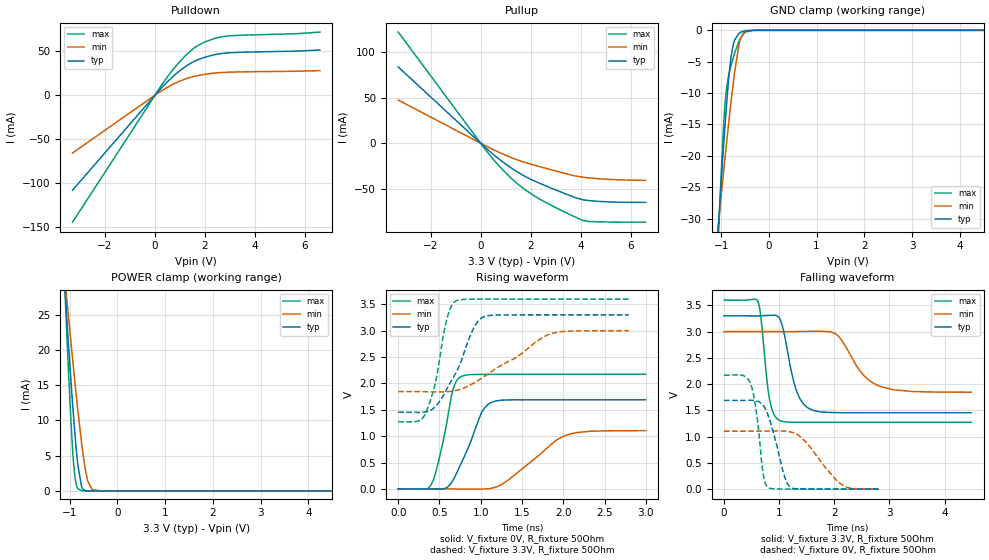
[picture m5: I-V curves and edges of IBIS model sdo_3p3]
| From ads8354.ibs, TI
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|   sdo_3p3 Model
[Model]   sdo_3p3
Model_type   3-state
Polarity   Non-Inverting
Vmeas = 1.65
Vref = 0
Cref = 10pF
Rref = 100
|   typ   min   max
|   (nom PVT)   (fast PVT)   (slow PVT)
C_comp   1.168e-12   9.199e-13   1.410e-12
| Where nom  PVT is Nominal Process, 3.3V, 27C
|   Fast PVT is Strong Process,  3.6V, -40C
|   Slow PVT is Weak Process,   3V, 125C
[Voltage Range]   3.3   3   3.6
|Junction Temperature
[Temperature Range]   27   125   -40
[Pullup Reference]   3.3   3   3.6
[Pulldown Reference]   0   0   0
[Power Clamp Reference]   3.3   3   3.6
[GND Clamp Reference]   0   0   0
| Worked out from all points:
|   slope of the pulldown table from 0 to 0.495 V, typ, clamps not added: 32.3 ohm
|   slope of the pullup table from 0 to 0.495 V, typ, clamps not added: 41.1 ohm
|   GND clamp passes 1 mA (typ) near -0.67 V on its own axis
|   POWER clamp passes 1 mA (typ) near -0.76 V on its own axis
|   falling waveform, V_fixture 3.3V, R_fixture 50Ohm: 20-80 % time 236ps typ, 455ps min, 138ps max; typ from 3.3 V to 1.45 V
|   rising waveform, V_fixture 0V, R_fixture 50Ohm: 20-80 % time 266ps typ, 510ps min, 168ps max; typ from 0 V to 1.69 V
|   rising waveform, V_fixture 3.3V, R_fixture 50Ohm: 20-80 % time 314ps typ, 664ps min, 173ps max; typ from 1.45 V to 3.3 V
|   falling waveform, V_fixture 0V, R_fixture 50Ohm: 20-80 % time 253ps typ, 496ps min, 146ps max; typ from 1.69 V to 0 V
[Pulldown]
|   Voltage   I(typ)   I(min)   I(max)
-3.3V     -108.3mA   -65.93mA   -144.9mA
276mV     8.889mA    5.263mA    12.04mA
580.8mV   17.73mA    10.37mA    24.11mA
922.8mV   26.37mA    15.19mA    36.09mA
1.254V    33.38mA    18.88mA    46.05mA
1.582V    38.81mA    21.55mA    54.12mA
1.833V    41.77mA    23.03mA    58.51mA
2.262V    45.4mA     24.87mA    63.57mA
2.835V    48.1mA     26.13mA    67.38mA
5.702V    50.35mA    27.36mA    70.25mA
6.6V      51.63mA    28.07mA    72.02mA
[GND Clamp]
|   Voltage   I(typ)   I(min)   I(max)
-3.3V     -330.2mA   -221.1mA   -504.8mA
-1.063V   -31.82mA   -31.36mA   -34mA
-1.01V    -25.58mA   -27.31mA   -24.71mA
-943.8mV  -17.95mA   -22.25mA   -14.61mA
-921mV    -15.46mA   -20.55mA   -12mA
-881.1mV  -11.36mA   -17.62mA   -8.898mA
-788.7mV  -4.041mA   -11.17mA   -5.539mA
-745.8mV  -2.266mA   -8.406mA   -4.364mA
-624mV    -483.8uA   -2.208mA   -1.712mA
-528mV    -102.4uA   -293.2uA   -540.5uA
-306mV    -437.8nA   -899.4nA   -2.577uA
6.6V      0A         0A         0A
[Pullup]
|   Voltage   I(typ)   I(min)   I(max)
-3.3V     83.61mA    47.33mA    121.8mA
300mV     -7.485mA   -4.247mA   -10.84mA
663.3mV   -15.8mA    -9.064mA   -22.63mA
1.052V    -23.85mA   -13.78mA   -33.91mA
1.647V    -34.34mA   -19.94mA   -48.25mA
2.439V    -44.79mA   -26.22mA   -62.42mA
3.789V    -59.57mA   -35.85mA   -80.89mA
4.116V    -62.05mA   -37.23mA   -84.72mA
4.3V      -62.7mA    -37.83mA   -85.66mA
5.488V    -64.6mA    -40.03mA   -86.46mA
6.6V      -64.75mA   -40.68mA   -86.47mA
[POWER Clamp]
|   Voltage   I(typ)   I(min)   I(max)
-3.3V     266.8mA    193.9mA    379.8mA
-1.158V   35.09mA    34.37mA    37.89mA
-1.054V   23.71mA    26.73mA    21.21mA
-970.8mV  15.33mA    20.89mA    9.481mA
-938.4mV  12.28mA    18.66mA    5.771mA
-904.2mV  9.237mA    16.34mA    2.838mA
-877.2mV  7.016mA    14.54mA    1.388mA
-831.6mV  3.796mA    11.6mA     344.4uA
-752.4mV  634.8uA    6.865mA    24.22uA
-624mV    6.907uA    1.455mA    326.5nA
-531mV    249.5nA    180uA      12.54nA
6.6V      0A         0A         0A
[Ramp]
R_load = 50
|   typ   min   max
dV/dt_r   1.01371/2.65885e-10   0.662544/5.07088e-10   1.30386/1.67243e-10
dV/dt_f   1.10733/2.33919e-10   0.692702/4.49517e-10   1.39661/1.37805e-10
[Falling Waveform]
V_fixture = 3.3V
V_fixture_min = 3V
V_fixture_max = 3.6V
R_fixture = 50Ohm
|   Time   V(typ)   V(min)   V(max)
0s        3.3V       3V         3.6V
609ps     3.298V     3V         3.596V
668.5ps   3.3V       3V         3.287V
826.5ps   3.31V      3V         1.714V
1.018ns   3.231V     3V         1.304V
1.311ns   1.884V     3.001V     1.273V
1.533ns   1.539V     3.006V     1.273V
2.025ns   1.458V     2.958V     1.273V
2.847ns   1.455V     1.95V      1.272V
4.485ns   1.454V     1.845V     1.272V
[Rising Waveform]
V_fixture = 0V
V_fixture_min = 0V
V_fixture_max = 0V
R_fixture = 50Ohm
|   Time   V(typ)   V(min)   V(max)
0s        3.043nV    8.004nV    3.91nV
334ps     -1.916mV   302.3uV    -5.453mV
399ps     -4.078mV   327.4uV    81.6mV
484ps     -5.087mV   110.7uV    492.2mV
670ps     180.1mV    -1.646mV   1.914V
762ps     482.5mV    -2.96mV    2.13V
1.015ns   1.458V     -2.846mV   2.171V
1.179ns   1.668V     31.42mV    2.172V
2.036ns   1.689V     1.018V     2.173V
2.998ns   1.69V      1.104V     2.173V
[Rising Waveform]
V_fixture = 3.3V
V_fixture_min = 3V
V_fixture_max = 3.6V
R_fixture = 50Ohm
|   Time   V(typ)   V(min)   V(max)
0s        1.454V     1.845V     1.272V
239.5ps   1.45V      1.846V     1.284V
332.5ps   1.46V      1.843V     1.437V
447.5ps   1.556V     1.839V     1.995V
591ps     1.899V     1.842V     3.235V
707.5ps   2.224V     1.87V      3.572V
912.5ps   3.045V     2.003V     3.598V
1.05ns    3.274V     2.14V      3.599V
1.839ns   3.299V     2.94V      3.6V
2.795ns   3.3V       3V         3.6V
[Falling Waveform]
V_fixture = 0V
V_fixture_min = 0V
V_fixture_max = 0V
R_fixture = 50Ohm
|   Time   V(typ)   V(min)   V(max)
0s        1.689V     1.104V     2.172V
482ps     1.694V     1.104V     2.012V
607ps     1.674V     1.104V     1.322V
715.5ps   1.592V     1.106V     267.1mV
807.5ps   1.387V     1.107V     24.14mV
1.066ns   357.7mV    1.107V     2.049mV
1.196ns   44.86mV    1.093V     1.013mV
1.484ns   3.685mV    901.9mV    582.8uV
2.142ns   480.5uV    80.23mV    197.2uV
2.803ns   199.1uV    3.02mV     67.19uV
